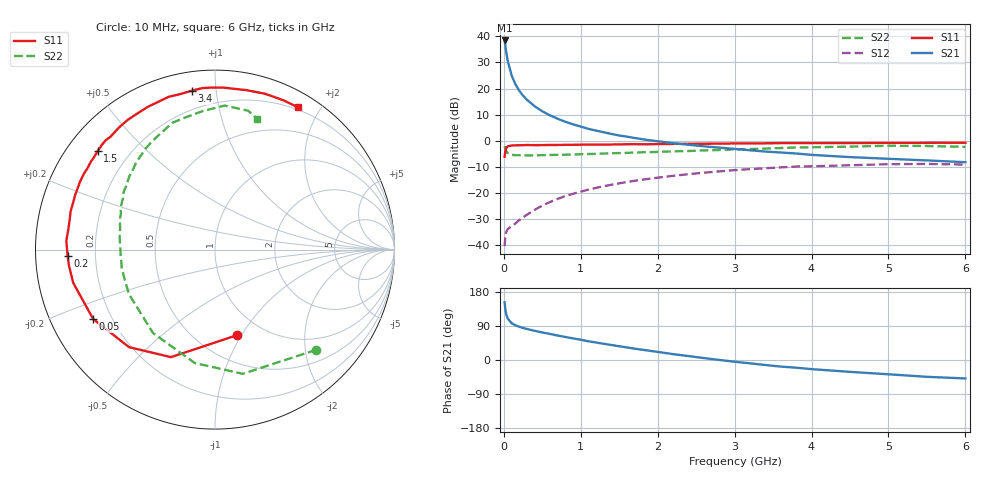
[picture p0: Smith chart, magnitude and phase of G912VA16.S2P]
! SIEMENS Small Signal Semiconductors
! BFG235
! Si NPN RF Bipolar Junction Transistor in SOT223
! VCE = 12 V  IC = 160 mA
! Common Emitter S-Parameters:  July  1994
# GHz  S  MA  R  50
!  f  S11  S21  S12  S22
! GHz  MAG  ANG  MAG  ANG  MAG  ANG  MAG  ANG
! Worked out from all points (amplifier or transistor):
!   40 points, 10 MHz to 6 GHz, reference 50 ohm
!   highest |S21| = 38.4 dB at 10 MHz (marker M1)
!   |S21| within 3 dB of that: start of sweep to 24.31 MHz
!   unconditionally stable (mu >= 1): 454.3 MHz to 1.514 GHz
!   at 200 MHz: K = 0.79, MSG = 24.8 dB, |S12| = -30.4 dB
!   at 1.5 GHz: K = 1.00, MAG = 8.9 dB, |S12| = -16.3 dB
!   at 6 GHz: K = 0.90, MSG = 0.5 dB, |S12| = -9.1 dB
!   S11 on the Smith chart (normalised r, x): 10 MHz: 0.76, -0.95; 50 MHz: 0.13, -0.26; 200 MHz: 0.10, -0.02; 1.5 GHz: 0.09, +0.36; 3.4 GHz: 0.10, +0.86; 6 GHz: 0.17, +1.73
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0.01  0.4925 -75.8  83.39 152.4  0.0096 61.8  0.7938 -44.7
0.02  0.6475 -112.3  65.53 133.5  0.015 47.8  0.709 -77.4
0.03  0.7244 -131.4  51.45 121.7  0.0177 41.0  0.642 -100.1
0.05  0.7812 -150.3  34.26 109.3  0.0204 33.4  0.5788 -126.7
0.1  0.8113 -166.8  18.08 97.3  0.023 35.8  0.54 -152.7
0.15  0.8185 -173.7  12.14 91.4  0.0261 41.9  0.5291 -163.5
0.2  0.8219 -177.5  9.088 87.7  0.0303 46.5  0.5293 -169.2
0.25  0.8252 179.2  7.317 84.5  0.0342 50.8  0.5261 -173.1
0.3  0.8299 176.6  6.113 82.0  0.0383 53.6  0.527 -176.3
0.4  0.8249 172.0  4.597 77.0  0.0477 57.1  0.5269 179.4
0.5  0.8266 168.3  3.671 72.6  0.0573 58.8  0.5308 176.0
0.6  0.8322 165.3  3.063 68.8  0.0673 59.5  0.535 172.9
0.7  0.8325 161.6  2.639 64.5  0.0773 59.6  0.5388 170.2
0.9  0.8379 156.0  2.066 57.0  0.0967 57.8  0.5465 165.6
1.1  0.8439 149.8  1.693 49.4  0.1162 55.4  0.5585 161.0
1.5  0.8532 140.0  1.263 36.2  0.1534 49.2  0.5823 152.7
2.2  0.8712 124.0  0.903 15.5  0.2133 36.8  0.6278 139.5
3.2  0.8878 102.6  0.659 -8.8  0.2865 17.5  0.6956 120.7
3.4  0.8947 98.4  0.622 -13.2  0.2981 13.5  0.7101 116.4
4.5  0.9056 78.7  0.487 -31.3  0.34 -7.4  0.7735 95.5
5.5  0.9148 65.5  0.421 -44.4  0.3604 -25.8  0.7957 76.6
6  0.9184 59.6  0.389 -48.7  0.3505 -32.5  0.7649 72.0
